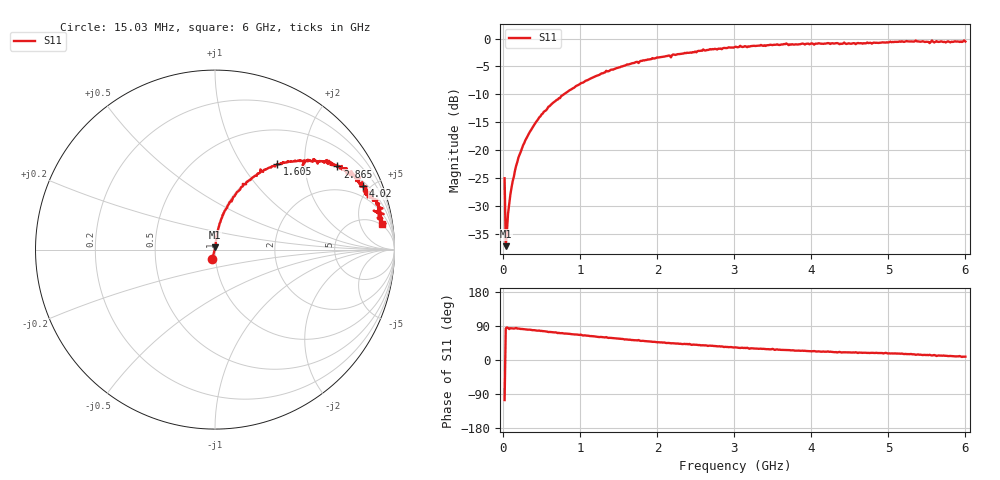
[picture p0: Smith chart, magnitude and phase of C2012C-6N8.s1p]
!	Network	Analyzer	HP8753E.07.74:	Oct	30	2002	Serial	No.	JP38451487
!	Hewlett-Packard
!	7	Sep	2009	10:41:17
!	Frequency	S11
#	HZ	S	RI	R	50
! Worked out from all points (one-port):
!   400 points, 15.03 MHz to 6 GHz, reference 50 ohm
!   lowest |S11| = -37.3 dB at 30.03 MHz (marker M1), VSWR 1.03, Z = 50.1 + j1.36 ohm
!   |S11| at or under -10 dB: start of sweep to 784.4 MHz
!   S11 on the Smith chart (normalised r, x): 15.03 MHz: 0.96, -0.10; 1.605 GHz: 1.00, +1.45; 2.865 GHz: 1.02, +2.94; 4.02 GHz: 1.23, +4.53; 6 GHz: 4, +11
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1.502992e7  -0.0151 -0.0536
3.002985e7  0.00154 0.0136
6.00297e7  0.00268 0.0268
9.002955e7  0.0043 0.0396
1.95029e8  0.0105 0.0851
2.850286e8  0.0198 0.121
4.650277e8  0.0413 0.192
7.650262e8  0.101 0.292
1.335023e9  0.253 0.447
1.515022e9  0.312 0.457
1.605022e9  0.345 0.475
2.265019e9  0.526 0.499
2.865016e9  0.682 0.463
3.015015e9  0.707 0.466
3.195014e9  0.736 0.419
3.495013e9  0.761 0.43
3.525012e9  0.786 0.394
3.555012e9  0.784 0.418
3.765011e9  0.797 0.381
4.02001e9  0.825 0.355
4.515007e9  0.845 0.306
5.265004e9  0.908 0.25
5.355003e9  0.933 0.229
5.535002e9  0.884 0.217
5.565002e9  0.94 0.198
5.595002e9  0.899 0.209
5.625002e9  0.932 0.173
6e9  0.93 0.144
